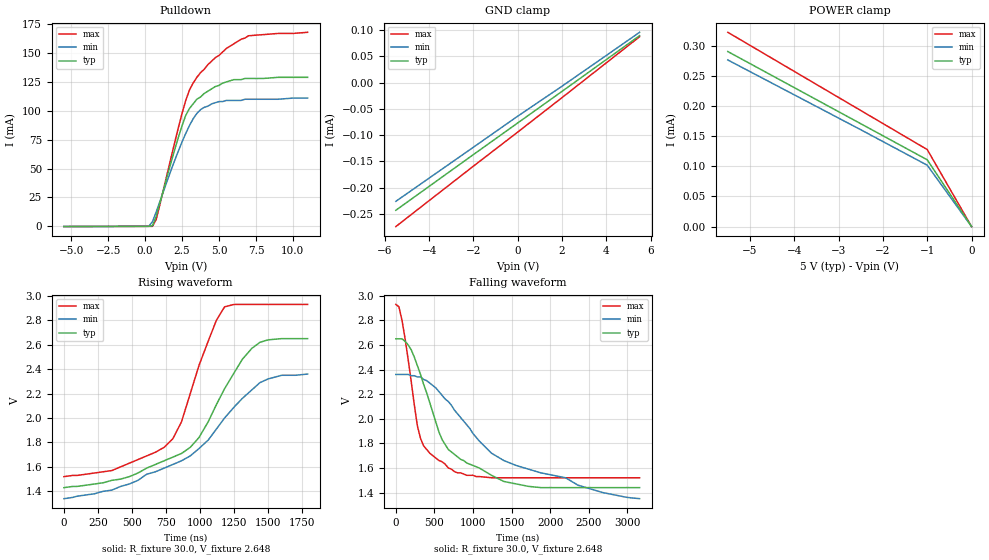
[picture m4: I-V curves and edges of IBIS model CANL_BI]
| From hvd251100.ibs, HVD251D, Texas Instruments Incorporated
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|   Driver (CANL) Output/Receiver Input Model
[Model]   CANL_BI
Model_type   I/O_open_drain
| Signals   CANH
Vinh = 0.9V
Vinl = 0.5V
Rref = 30   |Note: 60 Ohm differential load;
Vref = 2.3   |tr, tf measured in single ended configuration
| variable   typ   min   max
C_comp   1.0pF   NA   NA
|   typ   min   max
[Temperature Range]   25.0   -40   125
[Voltage Range]   5.0V   4.5V   5.5V
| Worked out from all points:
|   slope of the pulldown table from 0 to 0.75 V, typ, clamps not added: 84.4 ohm
|   rising waveform, R_fixture 30.0, V_fixture 2.648: 20-80 % time 482ns typ, 686ns min, 292ns max; typ from 1.43 V to 2.65 V
|   falling waveform, R_fixture 30.0, V_fixture 2.648: 20-80 % time 523ns typ, 1.3us min, 225ns max; typ from 2.65 V to 1.44 V
[Pulldown]
|   Voltage   I(typ)   I(min)   I(max)
-5.5V     -243uA     -226uA     -274uA
250mV     -72.3uA    20.6uA     -87.7uA
500mV     382uA      4.06mA     -72.2uA
750mV     8.81mA     12.4mA     5.92mA
2.5V      87.1mA     73.1mA     97.8mA
3V        102mA      87.2mA     118mA
3.5V      110mA      97.7mA     129mA
4V        115mA      103mA      136mA
5V        122mA      108mA      148mA
6V        127mA      109mA      158mA
7V        128mA      110mA      165mA
11V       129mA      111mA      168mA
[Power_clamp]
| Note that the[POWER_clamp]voltage table is referenced to Vcc
| and is calculated using Vtable=Vcc - Vmeasured.
|   Voltage   I(typ)   I(min)   I(max)
-5.5V     291uA      277uA      323uA
-4V       231uA      219uA      258uA
-2.5V     171uA      161uA      193uA
-1V       111uA      102uA      128uA
0V        0A         0A         0A
[GND_clamp]
|   Voltage   I(typ)   I(min)   I(max)
-5.5V     -243uA     -226uA     -274uA
-2V       -137uA     -123uA     -159uA
0V        -76.8uA    -63.9uA    -94.2uA
2V        -16.7uA    -6.87uA    -28.6uA
5.5V      89.3uA     95.7uA     87.3uA
[Ramp]
|   typ   min   max
dV/dt_r   1.22/800ns   1.02/992ns   1.41/576ns
dV/dt_f   1.21/980ns   1.01/1900ns   1.41/480ns
R_load = 30ohm  | Note: The measurement is single-ended with 30ohm
|   to Vfixture
[Rising Waveform]
R_fixture = 30.0
V_fixture = 2.648
V_fixture_min = 2.356
V_fixture_max = 2.927
C_fixture = 0p
L_fixture = 0n
|   V(typ)   V(min)   V(max)
0s        1.43V      1.34V      1.52V
352ns     1.49V      1.41V      1.57V
800ns     1.68V      1.62V      1.83V
864ns     1.71V      1.65V      1.97V
992ns     1.84V      1.75V      2.43V
1.12us    2.11V      1.91V      2.8V
1.18us    2.24V      2V         2.91V
1.31us    2.48V      2.16V      2.93V
1.44us    2.62V      2.29V      2.93V
1.79us    2.65V      2.36V      2.93V
[Falling Waveform]
R_fixture = 30.0
V_fixture = 2.648
V_fixture_min = 2.356
V_fixture_max = 2.927
C_fixture = 0p
L_fixture = 0n
|   V(typ)   V(min)   V(max)
0s        2.65V      2.36V      2.93V
40ns      2.65V      2.36V      2.91V
80ns      2.65V      2.36V      2.8V
280ns     2.43V      2.34V      1.94V
320ns     2.36V      2.34V      1.84V
560ns     1.89V      2.22V      1.66V
680ns     1.75V      2.14V      1.6V
1.08us    1.6V       1.82V      1.53V
1.4us     1.49V      1.66V      1.52V
3.16us    1.44V      1.35V      1.52V
